|   Package Model For TMS570LS09x/07xPZ
[IBIS Ver]   4.1
[File Name]   tms570ls09x_07x_pz.ibs
[File Rev]   1.0
[Date]   Thu Sep 4 18:41:18 2014
[Source]   Texas Instruments, Inc.
[Notes]   Revision History:
   1.0: initial release, 09/04/2014
   THIS IS RELEASE 1.0,THE CONTENTS ARE SUBJECT TO
   CHANGE WITHOUT PRIOR NOTICE,IF NECESSARY.
[Disclaimer] Please be aware that in the absence of a written agreement
   Texas Instruments(TI) assumes no liability for:
   (1) The accuracy of the IBIS models provided to your company
   (2) The proper functioning of these Models in your design
   or for any resulting applications;or
   (3) Infringement of patents,copyrights or intellectual
   property rights resulting from your use of these models.
   TI provides IBIS Models as a service to our customers and
   therefore reserves the right to limit distribution of the
   Models.
[Copyright]   Property of Texas Instruments Incorporated.
   Unauthorised reproduction and/or distribution is strictly.
   prohibited.
   This product is protected under copyright law and trade
   secret law as an unpublished work.
   Created 2013,(C) Copyright 2013-2014,
   Texas Instruments Incorporated., All Rights Reserved.
   These commodities are under the U.S. Government
   distribution license control.As such,they are not to be
   re-exported without the prior approval of the
   U.S. Department of Commerce.
[Component]   TMS570LS09x/07xPZ
[Manufacturer]   Texas Instruments
[Package]
| variable   typ   min   max
R_pkg   181.781m   70.1162m   236.912m
L_pkg   3.42482nH   2.25859nH   4.37162nH
C_pkg   0.353239pF   0.282584pF   0.478604pF
[Pin]   signal_name   model_name   R_pin   L_pin   C_pin
1	GIOA[0]	BQ0210FS_PD_3X2	219.723m	4.04947nH	0.322214pF
2	GIOA[1]	BQ0210FS_PD_3X2	216.923m	4.00487nH	0.359891pF
|3	FLTP1	TP1_220UM	211.298m	3.88259nH	0.355891pF
|4	FLTP2	BAFTHRU8VFT	207.257m	3.79631nH	0.348827pF
5	GIOA[2]	BQ0215FS_PD_3X2	212.445m	3.91729nH	0.345709pF
|6	VCCIO	0	116.048m	3.34405nH	0.395737pF
|7	VSS	0	210.61m	3.85025nH	0.355502pF
8	GIOA[3]	BQ0210FS_PD_3X2	206.124m	3.78772nH	0.337599pF
9	GIOA[4]	BQ0210FS_PD_3X2	209.49m	3.86735nH	0.337949pF
10	GIOA[5]	BQ0215FS_PD_3X2	207.253m	3.79417nH	0.35504pF
11	NHET1[22]	BQ0215FS_PD_3X2	204.603m	3.70566nH	0.359508pF
12	GIOA[6]	BQ0215FS_PD_3X2	203.4m	3.64587nH	0.356722pF
|13	VCC	0	78.2164m	2.7409nH	0.433715pF
|14	OSCIN	0	200.842m	3.62846nH	0.33298pF
|15	KELVIN_GND	0	199.908m	3.61707nH	0.344537pF
|16	OSCOUT	0	201.796m	3.65406nH	0.3511pF
|17	VSS	0	108.948m	3.04442nH	0.396378pF
18	GIOA[7]	BQ0215FS_PD_3X2	201.042m	3.62877nH	0.338671pF
19	NHET1[0]	BQ0215FS_PD_3X2	201.752m	3.65877nH	0.335885pF
|20	VSS	0	109.665m	3.03407nH	0.411989pF
|21	VCC	0	79.2477m	2.771nH	0.478604pF
22	NHET1[02]	BQ0215FS_PD_3X2	211.962m	3.81885nH	0.377507pF
23	SPI2NCS[0]	BQ0210FS_PU_3X2	214.225m	3.91916nH	0.366651pF
24	TEST	BQ0213FS_PD_3X2	217.148m	4.01178nH	0.3756pF
25	NHET1[04]	BQ0215FS_PD_3X2	224.417m	4.16091nH	0.332095pF
26	NHET1[06]	BQ0215FS_PD_3X2	211.561m	3.83658nH	0.321795pF
27	MIBSPI1NCS[2]	BQ0215FS_PU_3X2	205.185m	3.69268nH	0.370932pF
|28	VCCIO	0	197.628m	3.50545nH	0.372961pF
|29	VSS	0	104.003m	2.82711nH	0.416032pF
|30	VCC	0	75.2232m	2.47926nH	0.437312pF
31	nPORRST	IQ0087FS_3X2	181.883m	3.11957nH	0.340105pF
|32	VCC	0	70.1162m	2.25859nH	0.419563pF
|33	VSS	0	177.617m	3.03415nH	0.327076pF
34	MIBSPI3SOMI	BT3304BHYPU_AICLN_3X2SF	171.937m	3.00185nH	0.305876pF
35	MIBSPI3SIMO	BT3304BHYPU_AICLN_3X2SF	170.478m	2.98577nH	0.309908pF
36	MIBSPI3CLK	BT3304BHYPU_AICLN_3X2SF	169.285m	2.9505nH	0.315789pF
37	MIBSPI3NENA	BQ0210FS_PU_3X2	168.876m	2.93664nH	0.314152pF
38	MIBSPI3NCS[0]	BQ0215FS_PU_3X2	169.754m	2.9666nH	0.309022pF
39	MIBSPI1NCS[3]	BQ0210FS_PU_3X2	167.85m	2.95402nH	0.282584pF
|40	AD1IN[16]_AD2IN[0]	ARCHER_ADC	163.366m	2.85111nH	0.298869pF
|41	AD1IN[17]_AD2IN[01]	ARCHER_ADC	165.138m	2.87865nH	0.315354pF
|42	AD1IN[0]	ARCHER_ADC	168.408m	2.93609nH	0.322537pF
|43	AD1IN[07]	ARCHER_ADC	173.147m	3.03087nH	0.319884pF
|44	AD1IN[20]_AD2IN[04]	ARCHER_ADC	175.267m	3.03792nH	0.32485pF
|45	AD1IN[21]_AD2IN[05]	ARCHER_ADC	184.451m	3.16402nH	0.348406pF
|46	ADREFHI	ARCHER_ADC	102.848m	2.7095nH	0.409628pF
|47	ADREFLO	0	103.128m	2.77224nH	0.402436pF
|48	AD1IN[09]_AD2IN[09]	ARCHER_ADC	196.065m	3.45571nH	0.371233pF
|49	AD1IN[01]	ARCHER_ADC	208.006m	3.71073nH	0.400905pF
|50	AD1IN[10]_AD2IN[10]	ARCHER_ADC	221.883m	4.03864nH	0.361798pF
|51	AD1IN[02]	ARCHER_ADC	236.912m	4.37162nH	0.375768pF
|52	AD1IN[03]	ARCHER_ADC	224.255m	4.10576nH	0.423224pF
|53	AD1IN[11]_AD2IN[11]	ARCHER_ADC	211.371m	3.86683nH	0.381547pF
|54	AD1IN[04]	ARCHER_ADC	192.903m	3.48836nH	0.337595pF
|55	AD1IN[05]	ARCHER_ADC	192.659m	3.47623nH	0.336519pF
|56	AD1IN[06]	ARCHER_ADC	192.888m	3.48803nH	0.330426pF
|57	AD1IN[08]_AD2IN[08]	ARCHER_ADC	193.032m	3.4996nH	0.316017pF
58	AD1EVT	BQ0210FS_PD_3X2	198.161m	3.59014nH	0.325956pF
|59	VSS	0	105.306m	2.9616nH	0.387788pF
|60	VCCIO	0	203.137m	3.58879nH	0.353218pF
|61	VCC	0	76.4981m	2.65477nH	0.447673pF
62	CAN1TX	BQ0210FS_PU_3X2	202.032m	3.65593nH	0.346952pF
63	CAN1RX	BQ0210FS_PU_3X2	204.775m	3.717nH	0.363947pF
64	NHET1[24]	BQ0210FS_PD_3X2	208.287m	3.81266nH	0.345107pF
65	MIBSPI1SIMO	BT3304BHYPU_AICLN_3X2SF	207.545m	3.79341nH	0.346331pF
66	MIBSPI1SOMI	BT3304BHYPU_AICLN_3X2SF	212.493m	3.88805nH	0.350646pF
67	MIBSPI1CLK	BT3304BHYPU_AICLN_3X2SF	211.543m	3.8907nH	0.354316pF
68	MIBSPI1NENA	BQ0215FS_PU_3X2	217.873m	4.02173nH	0.35955pF
69	SPI2SOMI	BQ0215FS_PU_3X2	214.986m	3.9908nH	0.338139pF
70	SPI2SIMO	BQ0215FS_PU_3X2	212.636m	3.92849nH	0.344025pF
71	SPI2CLK	BQ0215FS_PU_3X2	215.578m	3.96674nH	0.347035pF
|72	VSS	0	109.822m	2.98745nH	0.404779pF
73	MIBSPI1NCS[0]	BQ0215FS_PU_3X2	211.125m	3.87375nH	0.374496pF
74	NHET1[08]	BQ0215FS_PD_3X2	218.945m	4.04457nH	0.38818pF
75	TMS	BT3308BHYPP_AIC_3X2SF	225.88m	4.19379nH	0.333718pF
76	nTRST	IQ0087FS_3X2	215.753m	3.93723nH	0.340338pF
77	TDI	BQ0192FS_PU_3X2	203.763m	3.64913nH	0.389338pF
78	TDO	BT3308BHYPP_AIC_3X2SF	192.796m	3.42759nH	0.370918pF
79	TCK	IQ0079FS_PD_3X2	183.863m	3.23504nH	0.353162pF
80	RTCK	BT3308BHYPP_AIC_3X2SF	176.514m	3.09346nH	0.325544pF
81	nRST	BT3304BHYPD_AICDL_3X2SF	178.579m	3.18029nH	0.323687pF
82	nERROR	BT3308BHYPP_AIC_3X2SF	173.454m	3.05448nH	0.329573pF
83	NHET1[10]	BQ0215FS_PD_3X2	169.783m	2.98124nH	0.32307pF
84	ECLK	BQ0215FS_PD_3X2	167.838m	2.93748nH	0.316585pF
|85	VCCIO	0	167.255m	2.9215nH	0.31525pF
|86	VSS	0	168.393m	2.94969nH	0.315526pF
|87	VSS	0	170.832m	2.99538nH	0.317889pF
|88	VCC	0	174.675m	3.07628nH	0.330386pF
89	NHET1[12]	BQ0210FS_PD_3X2	179.632m	3.17094nH	0.329008pF
90	NHET1[14]	BQ0215FS_PD_3X2	185.11m	3.3116nH	0.321367pF
91	CAN2TX	BQ0210FS_PU_3X2	182.398m	3.25817nH	0.303229pF
92	CAN2RX	BQ0210FS_PU_3X2	178.742m	3.17539nH	0.320508pF
93	MIBSPI1NCS[1]	BQ0215FS_PU_3X2	185.805m	3.31999nH	0.337306pF
94	LINRX	BQ0210FS_PU_3X2	191.013m	3.40717nH	0.347232pF
95	LINTX	BQ0210FS_PU_3X2	201.223m	3.56318nH	0.359056pF
|96	VCCP	0	74.6547m	2.53914nH	0.416387pF
97	NHET1[16]	BQ0215FS_PD_3X2	182.634m	3.2498nH	0.337644pF
98	NHET1[18]	BQ0215FS_PD_3X2	191.497m	3.43782nH	0.356089pF
|99	VCC	0	195.593m	3.51404nH	0.370518pF
|100	VSS	0	208.181m	3.77143nH	0.33608pF
[Model Selector] BQ0192FS_PU_3X2
BQ0192FS_PU_3X2_PZ_3P3  Cell operated at 3.3(nom)
|BQ0192FS_PU_3X2_PZ_3P3; PUPD_OFF
BQ0192FS_PU_3X2_PU_3P3  Cell operated at 3.3(nom)
|BQ0192FS_PU_3X2_PU_3P3; PULLUP_ON
BQ0192FS_PU_3X2_PD_3P3  Cell operated at 3.3(nom)
|BQ0192FS_PU_3X2_PD_3P3; PULLDOWN_ON
[Model Selector] BQ0210FS_PU_3X2
BQ0210FS_PU_3X2_PZ_3P3  Cell operated at 3.3(nom)
|BQ0210FS_PU_3X2_PZ_3P3; PUPD_OFF
BQ0210FS_PU_3X2_PU_3P3  Cell operated at 3.3(nom)
|BQ0210FS_PU_3X2_PU_3P3; PULLUP_ON
BQ0210FS_PU_3X2_PD_3P3  Cell operated at 3.3(nom)
|BQ0210FS_PU_3X2_PD_3P3; PULLDOWN_ON
[Model Selector] BQ0210FS_PD_3X2
BQ0210FS_PD_3X2_PZ_3P3  Cell operated at 3.3(nom)
|BQ0210FS_PD_3X2_PZ_3P3; PUPD_OFF
BQ0210FS_PD_3X2_PU_3P3  Cell operated at 3.3(nom)
|BQ0210FS_PD_3X2_PU_3P3; PULLUP_ON
BQ0210FS_PD_3X2_PD_3P3  Cell operated at 3.3(nom)
|BQ0210FS_PD_3X2_PD_3P3; PULLDOWN_ON
[Model Selector] BQ0213FS_PD_3X2
BQ0213FS_PD_3X2_PD_3P3  Cell operated at 3.3(nom)
|BQ0213FS_PD_3X2_PD_3P3; PULLDOWN_ON
BQ0213FS_PD_3X2_PZ_3P3  Cell operated at 3.3(nom)
|BQ0213FS_PD_3X2_PZ_3P3; PULLUP_OFF
[Model Selector] BQ0215FS_PD_3X2
BQ0215FS_PD_3X2_PZ_3P3  Cell operated at 3.3(nom)
|BQ0215FS_PD_3X2_PZ_3P3; PUPD_OFF
BQ0215FS_PD_3X2_PU_3P3  Cell operated at 3.3(nom)
|BQ0215FS_PD_3X2_PU_3P3; PULLUP_ON
BQ0215FS_PD_3X2_PD_3P3  Cell operated at 3.3(nom)
|BQ0215FS_PD_3X2_PD_3P3; PULLDOWN_ON
[Model Selector] BQ0215FS_PU_3X2
BQ0215FS_PU_3X2_PZ_3P3  Cell operated at 3.3(nom)
|BQ0215FS_PU_3X2_PZ_3P3; PUPD_OFF
BQ0215FS_PU_3X2_PU_3P3  Cell operated at 3.3(nom)
|BQ0215FS_PU_3X2_PU_3P3; PULLUP_ON
BQ0215FS_PU_3X2_PD_3P3  Cell operated at 3.3(nom)
|BQ0215FS_PU_3X2_PD_3P3; PULLDOWN_ON
[Model Selector] BT3304BHYPD_AICDL_3X2SF
BT3304BHYPD_AICDL_3X2SF_PZ_3P3  Cell operated at 3.3(nom)
|BT3304BHYPD_AICDL_3X2SF_PZ_3P3; PUPD_OFF
BT3304BHYPD_AICDL_3X2SF_PU_3P3  Cell operated at 3.3(nom)
|BT3304BHYPD_AICDL_3X2SF_PU_3P3; PULLUP_ON
BT3304BHYPD_AICDL_3X2SF_PD_3P3  Cell operated at 3.3(nom)
|BT3304BHYPD_AICDL_3X2SF_PD_3P3; PULLDOWN_ON
[Model Selector] BT3304BHYPU_AICLN_3X2SF
BT3304BHYPU_AICLN_3X2SF_PZ_3P3  Cell operated at 3.3(nom)
|BT3304BHYPU_AICLN_3X2SF_PZ_3P3; PUPD_OFF
BT3304BHYPU_AICLN_3X2SF_PU_3P3  Cell operated at 3.3(nom)
|BT3304BHYPU_AICLN_3X2SF_PU_3P3; PULLUP_ON
BT3304BHYPU_AICLN_3X2SF_PD_3P3  Cell operated at 3.3(nom)
|BT3304BHYPU_AICLN_3X2SF_PD_3P3; PULLDOWN_ON
[Model Selector] BT3308BHYPP_AIC_3X2SF
BT3308BHYPP_AIC_3X2SF_PZ_3P3  Cell operated at 3.3(nom)
|BT3308BHYPP_AIC_3X2SF_PZ_3P3; PUPD_OFF
BT3308BHYPP_AIC_3X2SF_PU_3P3  Cell operated at 3.3(nom)
|BT3308BHYPP_AIC_3X2SF_PU_3P3; PULLUP_ON
BT3308BHYPP_AIC_3X2SF_PD_3P3  Cell operated at 3.3(nom)
|BT3308BHYPP_AIC_3X2SF_PD_3P3; PULLDOWN_ON
[Model Selector] IQ0079FS_PD_3X2
079FS_PD_3X2_3P3  Cell operated at 3.3(nom)
|IQ0079FS_PD_3X2_3P3; PUPD_OFF
FS_PD_3X2_PU_3P3  Cell operated at 3.3(nom)
|IQ0079FS_PD_3X2_PU_3P3; PULLUP_ON
FS_PD_3X2_PD_3P3  Cell operated at 3.3(nom)
|IQ0079FS_PD_3X2_PD_3P3; PULLDOWN_ON
[Model Selector] IQ0087FS_3X2
087FS_3X2_PD_3P3  Cell operated at 3.3(nom)
|IQ0087FS_3X2_PD_3P3; PULLDOWN_ON
IQ0087FS_3X2_3P3  Cell operated at 3.3(nom)
| Models and submodels in the file (31): BQ0192FS_PU_3X2_PZ_3P3 (I/O), BQ0192FS_PU_3X2_PU_3P3 (I/O), BQ0192FS_PU_3X2_PD_3P3 (I/O), BQ0210FS_PU_3X2_PZ_3P3 (I/O), BQ0210FS_PU_3X2_PU_3P3 (I/O), BQ0210FS_PU_3X2_PD_3P3 (I/O), BQ0210FS_PD_3X2_PZ_3P3 (I/O), BQ0210FS_PD_3X2_PU_3P3 (I/O), BQ0210FS_PD_3X2_PD_3P3 (I/O), BQ0213FS_PD_3X2_PD_3P3 (I/O), BQ0213FS_PD_3X2_PZ_3P3 (I/O), BQ0215FS_PD_3X2_PZ_3P3 (I/O), BQ0215FS_PD_3X2_PU_3P3 (I/O), BQ0215FS_PD_3X2_PD_3P3 (I/O), BQ0215FS_PU_3X2_PZ_3P3 (I/O), BQ0215FS_PU_3X2_PU_3P3 (I/O), BQ0215FS_PU_3X2_PD_3P3 (I/O), BT3304BHYPD_AICDL_3X2SF_PZ_3P3 (I/O), BT3304BHYPD_AICDL_3X2SF_PU_3P3 (I/O), BT3304BHYPD_AICDL_3X2SF_PD_3P3 (I/O), BT3304BHYPU_AICLN_3X2SF_PZ_3P3 (I/O), BT3304BHYPU_AICLN_3X2SF_PU_3P3 (I/O), BT3304BHYPU_AICLN_3X2SF_PD_3P3 (I/O), BT3308BHYPP_AIC_3X2SF_PZ_3P3 (I/O), BT3308BHYPP_AIC_3X2SF_PU_3P3 (I/O), BT3308BHYPP_AIC_3X2SF_PD_3P3 (I/O), 079FS_PD_3X2_3P3 (Input), FS_PD_3X2_PU_3P3 (Input), FS_PD_3X2_PD_3P3 (Input), 087FS_3X2_PD_3P3 (Input), IQ0087FS_3X2_3P3 (Input)
